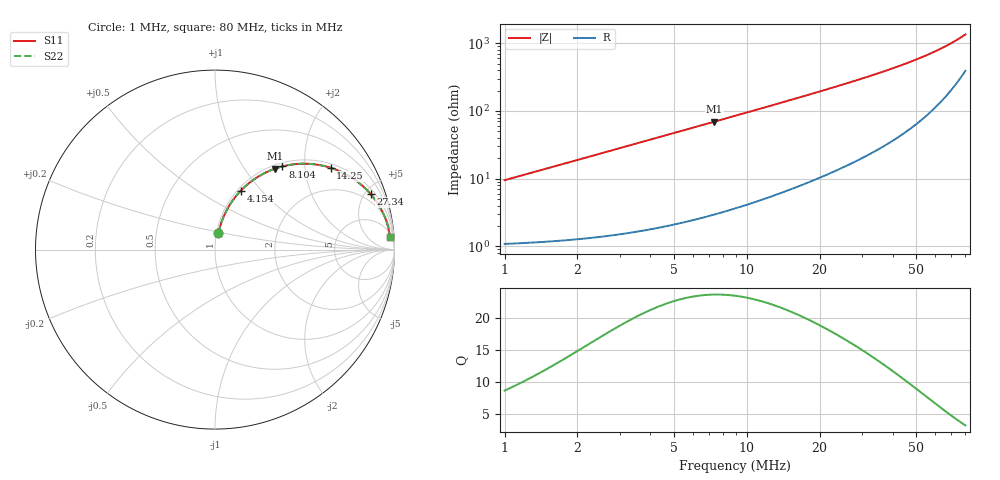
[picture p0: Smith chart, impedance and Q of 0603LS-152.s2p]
# MHz S MA R 50
!Freq  MagS11  AngS11  MagS21  AngS21  MagS12  AngS12  MagS22  AngS22
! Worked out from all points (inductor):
!   801 points, 1 MHz to 80 MHz, reference 50 ohm
!   read as one part in series: L = 1.5 uH near 1.022 MHz
!   highest Q = 23.6 at 7.344 MHz (marker M1), where L = 1.5 uH
!   S11 on the Smith chart (normalised r, x): 1 MHz: 1.02, +0.19; 4.154 MHz: 1.04, +0.78; 8.104 MHz: 1.07, +1.53; 14.25 MHz: 1.13, +2.72; 27.34 MHz: 1.34, +5.44; 80 MHz: 9, +26
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1  0.09344 78.1  0.985 -5.3  0.985 -5.3  0.09344 78.1
1.272536  0.1183 77.9  0.9819 -6.8  0.9819 -6.8  0.1183 77.9
1.549919  0.1433 77.2  0.9782 -8.2  0.9782 -8.2  0.1433 77.2
1.877453  0.1726 76.1  0.9729 -9.9  0.9729 -9.9  0.1726 76.1
2.237138  0.2041 74.7  0.9662 -11.8  0.9662 -11.8  0.2041 74.7
3.107596  0.2776 70.9  0.9463 -16.1  0.9463 -16.1  0.2776 70.9
4.154361  0.3595 66.3  0.9165 -21.0  0.9165 -21.0  0.3595 66.3
5.614896  0.4605 60.1  0.8679 -27.4  0.8679 -27.4  0.4605 60.1
7.343548  0.5597 53.6  0.8053 -34.0  0.8053 -34.0  0.5597 53.6
8.104486  0.5968 51.0  0.7775 -36.6  0.7775 -36.6  0.5968 51.0
11.13524  0.7116 42.2  0.6719 -45.3  0.6719 -45.3  0.7116 42.2
14.16999  0.7873 35.5  0.5809 -51.9  0.5809 -51.9  0.7873 35.5
14.24782  0.7888 35.3  0.5788 -52.0  0.5788 -52.0  0.7888 35.3
16.88469  0.8334 30.8  0.5129 -56.3  0.5129 -56.3  0.8334 30.8
19.90027  0.8694 26.7  0.4503 -60.2  0.4503 -60.2  0.8694 26.7
23.3263  0.8977 23.1  0.3922 -63.7  0.3922 -63.7  0.8977 23.1
27.34217  0.9203 19.7  0.3378 -66.7  0.3378 -66.7  0.9203 19.7
33.30213  0.9415 16.0  0.2759 -69.9  0.2759 -69.9  0.9415 16.0
40.56122  0.9566 12.7  0.2204 -72.4  0.2204 -72.4  0.9566 12.7
53.9277  0.9701 8.6  0.151 -74.3  0.151 -74.3  0.9701 8.6
67.13769  0.9753 5.9  0.1049 -73.4  0.1049 -73.4  0.9753 5.9
80  0.9766 4.0  0.07218 -69.1  0.07218 -69.1  0.9766 4.0
